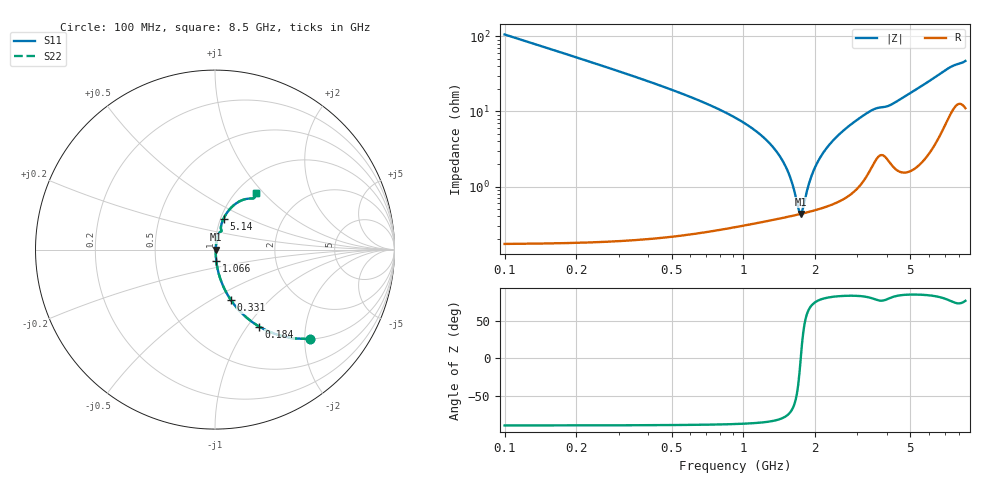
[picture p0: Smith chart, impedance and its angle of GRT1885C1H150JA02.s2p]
!Murata Part Number: GRT1885C1H150JA02
!These Parameters are Measured in Series Mode Connection
!Data Generated on Jun 19, 2026
!  o--ll--o
!Port1  Port2
!  o------o
!Operation Temp=25[degC], DC Bias Voltage=0[V]
!Freq. Start=100[MHz] Stop=9[GHz] 401[Steps]
# Hz S RI R 50
!Freq.(Hz) S11(Real) S11(Imag) S21(Real) S21(Imag) S12(Real) S12(Imag) S22(Real) S22(Imag)
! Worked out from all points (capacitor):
!   401 points, 100 MHz to 8.5 GHz, reference 50 ohm
!   read as one part in series: C = 15 pF near 142 MHz
!   lowest |Z| = 432 mohm at 1.738 GHz (marker M1)
!   series resonance near 1.738 GHz, so ESL is about 560 pH
!   S11 on the Smith chart (normalised r, x): 100 MHz: 1.00, -2.11; 184 MHz: 1.00, -1.14; 331 MHz: 1.00, -0.62; 1.066 GHz: 1.01, -0.12; 5.14 GHz: 1.03, +0.37; 8.5 GHz: 1.22, +0.91
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1e8  0.5279 -0.4984  0.4721 0.4984  0.4721 0.4984  0.5279 -0.4984
1.84e8  0.246 -0.4291  0.754 0.4291  0.754 0.4291  0.246 -0.4291
3.31e8  0.0885 -0.281  0.9115 0.281  0.9115 0.281  0.0885 -0.281
6.04e8  0.0254 -0.1501  0.9746 0.1501  0.9746 0.1501  0.0254 -0.1501
1.066e9  0.00694 -0.0616  0.9931 0.0616  0.9931 0.0616  0.00694 -0.0616
1.318e9  0.00473 -0.0342  0.9953 0.0342  0.9953 0.0342  0.00473 -0.0342
1.507e9  0.00419 -0.0175  0.9958 0.0175  0.9958 0.0175  0.00419 -0.0175
1.591e9  0.00415 -0.0109  0.9959 0.0109  0.9959 0.0109  0.00415 -0.0109
1.696e9  0.00423 -0.00301  0.9958 0.00301  0.9958 0.00301  0.00423 -0.00301
1.738e9  0.0043 5.4e-06  0.9957 -5.4e-06  0.9957 -5.4e-06  0.0043 5.4e-06
1.78e9  0.00438 0.00296  0.9956 -0.00296  0.9956 -0.00296  0.00438 0.00296
1.864e9  0.00461 0.00868  0.9954 -0.00868  0.9954 -0.00868  0.00461 0.00868
1.948e9  0.00491 0.0142  0.9951 -0.0142  0.9951 -0.0142  0.00491 0.0142
2.137e9  0.00581 0.0261  0.9942 -0.0261  0.9942 -0.0261  0.00581 0.0261
2.452e9  0.00805 0.0446  0.992 -0.0446  0.992 -0.0446  0.00805 0.0446
2.914e9  0.0136 0.0705  0.9864 -0.0705  0.9864 -0.0705  0.0136 0.0705
3.481e9  0.0288 0.0986  0.9712 -0.0986  0.9712 -0.0986  0.0288 0.0986
4.3e9  0.0328 0.1233  0.9672 -0.1233  0.9672 -0.1233  0.0328 0.1233
5.14e9  0.048 0.1732  0.952 -0.1732  0.952 -0.1732  0.048 0.1732
5.707e9  0.0682 0.2074  0.9318 -0.2074  0.9318 -0.2074  0.0682 0.2074
7.114e9  0.1617 0.2792  0.8383 -0.2792  0.8383 -0.2792  0.1617 0.2792
8.5e9  0.2297 0.3169  0.7703 -0.3169  0.7703 -0.3169  0.2297 0.3169
